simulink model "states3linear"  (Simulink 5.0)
settings: Solver=ode45  StartTime=0.0  StopTime=10  MaxStep=1e-3  RelTol=1e-3
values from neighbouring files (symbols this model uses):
  alpha0 = 3.77    [Load_Parameters.m]
  ap = -2.3    [Load_Parameters.m]
  B = 0.016033    [Load_Parameters.m]
  bp = 15369    [Load_Parameters.m]
  Gmp = 4.5e-9    (= 4.5e-09)    [Load_Parameters.m]
  Jc = 1.0472    [Load_Parameters.m]
  Mo = -2.08e-5    (= -2.08e-05)    [Load_Parameters.m]
  n0 = 800    [Load_Parameters.m]
  p0 = 24873    [Load_Parameters.m]
  T_p = 20    [Load_Parameters.m]
libraries: simulink_extras x1

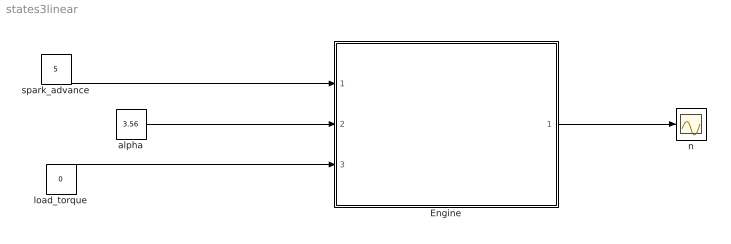
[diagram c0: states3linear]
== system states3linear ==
  Engine : Subsystem
  alpha : Constant  Value=3.56
  load_torque : Constant  Value=0
  n : Scope
  spark_advance : Constant  Value=5
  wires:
  Engine/1(Out1) -> n/1
  spark_advance/1 -> Engine/1(spark_advance)
  alpha/1 -> Engine/2(alpha)
  load_torque/1 -> Engine/3(load_torque)

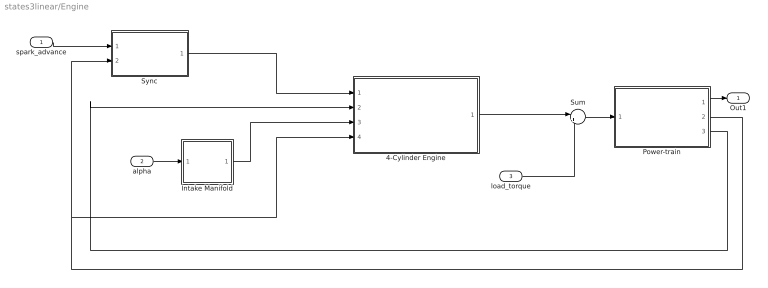
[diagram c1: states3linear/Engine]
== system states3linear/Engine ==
  spark_advance : Inport
  alpha : Inport  Port=2
  load_torque : Inport  Port=3
  4-Cylinder Engine : Subsystem
  Intake Manifold : Subsystem
  Power-train : Subsystem
  Sum : Sum  Inputs=|+-
  Sync : Subsystem
  Out1 : Outport
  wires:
  4-Cylinder Engine/1(T) -> Sum/1
  Power-train/2(theta) -> Sync/2(theta), 4-Cylinder Engine/4(theta)
  Sum/1 -> Power-train/1(T_eff)
  Sync/1(spark) -> 4-Cylinder Engine/1(spark)
  Power-train/3(DC) -> 4-Cylinder Engine/2(DC)
  Intake Manifold/1(m) -> 4-Cylinder Engine/3(m)
  load_torque/1 -> Sum/2
  spark_advance/1 -> Sync/1(spark_advance)
  alpha/1 -> Intake Manifold/1(alpha)
  Power-train/1(n) -> Out1/1

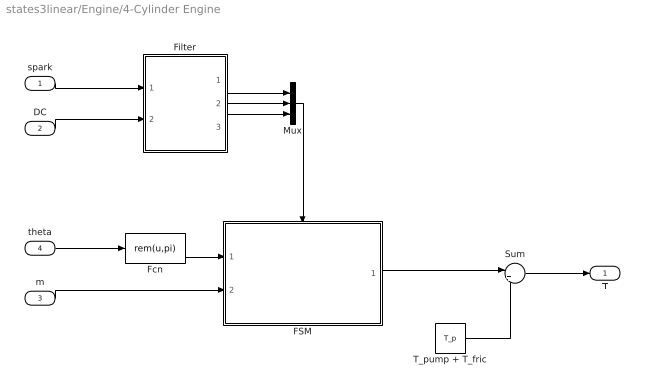
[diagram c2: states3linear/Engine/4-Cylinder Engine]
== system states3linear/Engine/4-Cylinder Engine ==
  spark : Inport
  DC : Inport  Port=2
  m : Inport  Port=3
  theta : Inport  Port=4
  FSM : Stateflow chart  TreatAsAtomicUnit=on
  Fcn : Fcn  Expr=rem(u,pi)
  Filter : Subsystem
  Mux : Mux  Inputs=3
  Sum : Sum  Inputs=|+-
  T_pump + T_fric : Constant  Value=T_p
  T : Outport
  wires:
  Mux/1 -> FSM/Trigger
  Filter/2(DC) -> Mux/2
  Filter/3(sparkDC) -> Mux/3
  Filter/1(spark) -> Mux/1
  theta/1 -> Fcn/1
  DC/1 -> Filter/2(DC_in)
  spark/1 -> Filter/1(spark_in)
  Fcn/1 -> FSM/1(theta)
  m/1 -> FSM/2(mc)
  Sum/1 -> T/1
  FSM/1(T_eff) -> Sum/1
  T_pump + T_fric/1 -> Sum/2

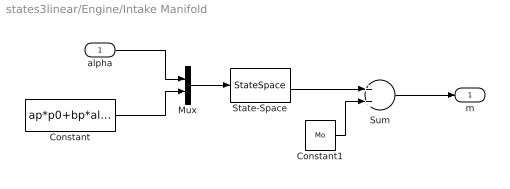
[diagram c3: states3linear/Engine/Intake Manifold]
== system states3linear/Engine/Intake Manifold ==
  alpha : Inport
  Constant : Constant  Value=ap*p0+bp*alpha0
  Constant1 : Constant  Value=Mo
  Mux : Mux  Inputs=2
  State-Space : StateSpace  A=ap  B=[bp -1]  C=Gmp  D=[0 0]  X0=p0
  Sum : Sum
  m : Outport
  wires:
  State-Space/1 -> Sum/1
  Mux/1 -> State-Space/1
  alpha/1 -> Mux/1
  Constant/1 -> Mux/2
  Sum/1 -> m/1
  Constant1/1 -> Sum/2

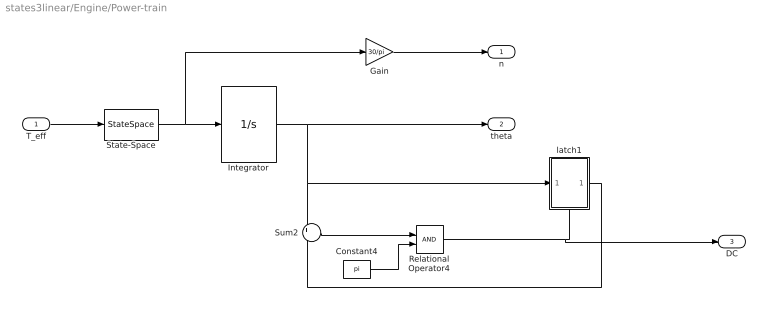
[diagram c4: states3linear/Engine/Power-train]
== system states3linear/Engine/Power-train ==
  T_eff : Inport
  Constant4 : Constant  Value=pi
  Gain : Gain  Gain=30/pi
  Integrator : Integrator
  Relational Operator4 : RelationalOperator
  State-Space : StateSpace  A=-B/Jc  B=1/Jc  D=0  X0=pi*n0/30
  Sum2 : Sum  Inputs=+-
  latch1 : Subsystem  TreatAsAtomicUnit=on
  n : Outport
  theta : Outport  Port=2
  DC : Outport  Port=3
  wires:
  T_eff/1 -> State-Space/1
  State-Space/1 -> Integrator/1, Gain/1
  Integrator/1 -> theta/1, latch1/1(In), Sum2/1
  latch1/1(Out) -> Sum2/2
  Sum2/1 -> Relational Operator4/1
  Constant4/1 -> Relational Operator4/2
  Relational Operator4/1 -> latch1/Trigger, DC/1
  Gain/1 -> n/1

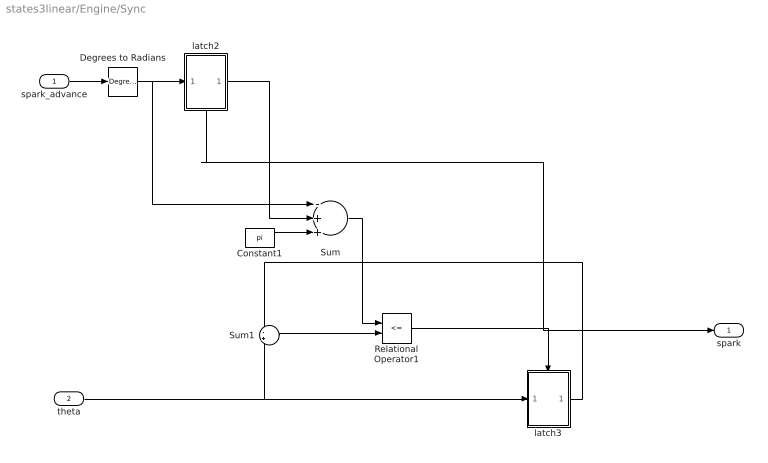
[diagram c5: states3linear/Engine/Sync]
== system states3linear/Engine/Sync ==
  spark_advance : Inport
  theta : Inport  Port=2
  Constant1 : Constant  Value=pi
  Degrees to Radians : simulink_extras/Transformations/Degrees to Radians
  Relational Operator1 : RelationalOperator  Operator=<=
  Sum : Sum  Inputs=-++
  Sum1 : Sum  Inputs=-+
  latch2 : Subsystem  TreatAsAtomicUnit=on
  latch3 : Subsystem  TreatAsAtomicUnit=on
  spark : Outport
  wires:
  latch2/1(Out) -> Sum/2
  Relational Operator1/1 -> latch3/Trigger, latch2/Trigger, spark/1
  Sum1/1 -> Relational Operator1/2
  latch3/1(Out) -> Sum1/1
  Sum/1 -> Relational Operator1/1
  Constant1/1 -> Sum/3
  theta/1 -> latch3/1(In), Sum1/2
  Degrees to Radians/1 -> latch2/1(In), Sum/1
  spark_advance/1 -> Degrees to Radians/1

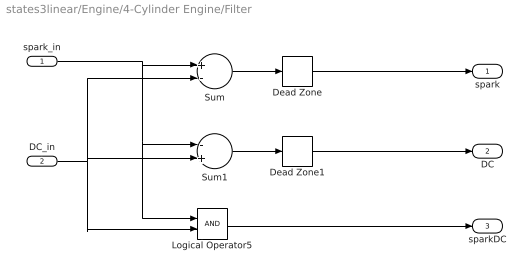
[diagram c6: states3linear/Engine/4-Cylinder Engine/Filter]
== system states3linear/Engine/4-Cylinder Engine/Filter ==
  spark_in : Inport
  DC_in : Inport  Port=2
  Dead Zone : DeadZone  LowerValue=-2  UpperValue=0
  Dead Zone1 : DeadZone  LowerValue=-2  UpperValue=0
  Logical Operator5 : Logic
  Sum : Sum  Inputs=+-
  Sum1 : Sum  Inputs=-+
  spark : Outport
  DC : Outport  Port=2
  sparkDC : Outport  Port=3
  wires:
  DC_in/1 -> Sum/2, Sum1/2, Logical Operator5/2
  Sum/1 -> Dead Zone/1
  Sum1/1 -> Dead Zone1/1
  spark_in/1 -> Sum/1, Sum1/1, Logical Operator5/1
  Dead Zone1/1 -> DC/1
  Dead Zone/1 -> spark/1
  Logical Operator5/1 -> sparkDC/1

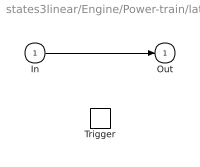
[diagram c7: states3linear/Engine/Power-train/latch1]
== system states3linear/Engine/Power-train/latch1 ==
  In : Inport
  Trigger : TriggerPort
  Out : Outport  InitialOutput=0
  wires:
  In/1 -> Out/1

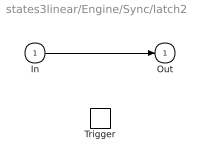
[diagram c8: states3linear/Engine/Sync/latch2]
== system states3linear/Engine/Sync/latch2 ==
  In : Inport
  Trigger : TriggerPort
  Out : Outport  InitialOutput=0
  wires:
  In/1 -> Out/1

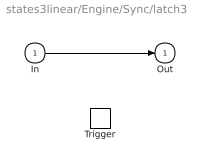
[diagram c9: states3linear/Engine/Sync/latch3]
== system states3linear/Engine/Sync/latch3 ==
  In : Inport
  Trigger : TriggerPort
  Out : Outport  InitialOutput=0
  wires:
  In/1 -> Out/1

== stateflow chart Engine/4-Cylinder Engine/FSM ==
  state Sl_minus
  state Sl
  state Sl_plus
  state eff = eta(ang) [function]
    (default) -> (junction 7) : {eff = eta_a + sqrt(eta_b+eta_c*ang);}
  Sl -> Sl_minus : dc/{me = mc;T_eff=0;}
  Sl_minus -> Sl : spark/{T_eff = (G*me+T0)*eta(-theta);}
  Sl -> Sl_plus : spark/{fi = pi-theta;}
  Sl_plus -> Sl : dc/{T_eff = (G*mc+T0)*eta(fi);}
  Sl -> Sl : sparkdc/{T_eff = (G*mc+T0)*eta(0);}
  (default) -> Sl
